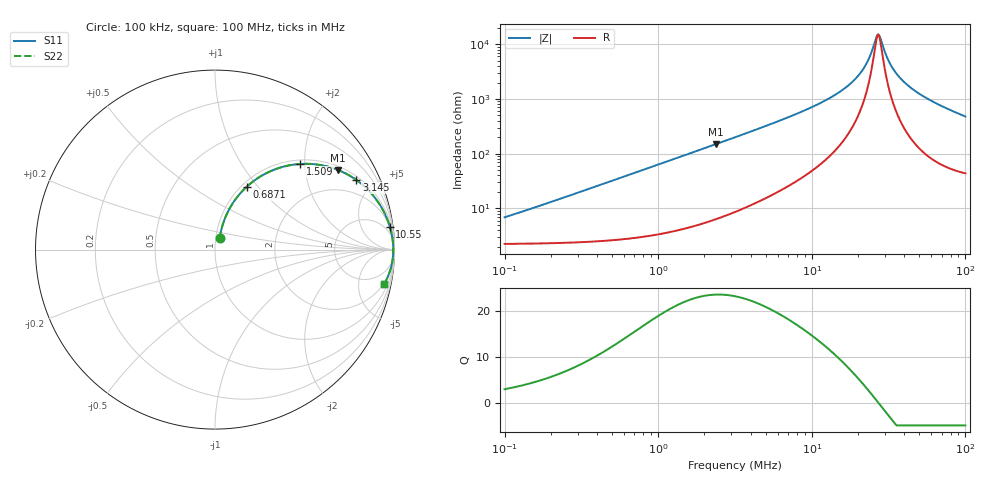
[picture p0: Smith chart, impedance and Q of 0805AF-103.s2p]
# MHz  S  MA  R  50
!Freq  MagS11  AngS11  MagS21  AngS21  MagS12  AngS12  MagS22  AngS22
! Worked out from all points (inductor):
!   801 points, 100 kHz to 100 MHz, reference 50 ohm
!   read as one part in series: L = 10.3 uH near 104.4 kHz
!   highest Q = 23.5 at 2.385 MHz (marker M1), where L = 10 uH
!   self-resonance near 27.05 MHz
!   S11 on the Smith chart (normalised r, x): 100 kHz: 1.04, +0.13; 687.1 kHz: 1.06, +0.87; 1.509 MHz: 1.09, +1.90; 3.145 MHz: 1.17, +3.96; 10.55 MHz: 2, +15; 100 MHz: 1.87, -9.53
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0.1  0.06706 67.3  0.9761 -3.6  0.9761 -3.6  0.06706 67.3
0.3183882  0.1965 72.0  0.9577 -11.3  0.9577 -11.3  0.1965 72.0
0.6870849  0.3908 63.3  0.8952 -23.0  0.8952 -23.0  0.3908 63.3
1.004987  0.5239 55.4  0.8246 -31.5  0.8246 -31.5  0.5239 55.4
1.508588  0.6737 45.1  0.7091 -42.3  0.7091 -42.3  0.6737 45.1
2.385071  0.8161 32.9  0.5442 -54.6  0.5442 -54.6  0.8161 32.9
3.144926  0.8777 26.3  0.4429 -61.3  0.4429 -61.3  0.8777 26.3
3.172224  0.8793 26.1  0.4399 -61.5  0.4399 -61.5  0.8793 26.1
5.282203  0.9467 16.2  0.2793 -71.0  0.2793 -71.0  0.9467 16.2
10.01307  0.981 7.9  0.1382 -78.2  0.1382 -78.2  0.981 7.9
10.546  0.9825 7.4  0.1292 -78.5  0.1292 -78.5  0.9825 7.4
15.29271  0.9897 4.1  0.07252 -79.8  0.07252 -79.8  0.9897 4.1
19.64868  0.9922 2.2  0.0398 -77.6  0.0398 -77.6  0.9922 2.2
22.95592  0.9931 1.1  0.02104 -70.2  0.02104 -70.2  0.9931 1.1
26.1334  0.9934 0.2  0.00783 -32.4  0.00783 -32.4  0.9934 0.2
26.81984  0.9934 0.1  0.006668 -9.4  0.006668 -9.4  0.9934 0.1
28.0042  0.9934 -0.2  0.007747 31.9  0.007747 31.9  0.9934 -0.2
31.88044  0.9932 -1.1  0.02093 70.5  0.02093 70.5  0.9932 -1.1
37.24652  0.9924 -2.2  0.03981 77.9  0.03981 77.9  0.9924 -2.2
46.63096  0.9901 -3.9  0.06929 79.8  0.06929 79.8  0.9901 -3.9
64.75956  0.9829 -6.8  0.1186 78.3  0.1186 78.3  0.9829 -6.8
100  0.9614 -11.5  0.2009 73.2  0.2009 73.2  0.9614 -11.5
